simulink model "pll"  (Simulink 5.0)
settings: Solver=ode4  StartTime=0.0  StopTime=5  FixedStep=0.001  RelTol=1e-6
libraries: simulink x1

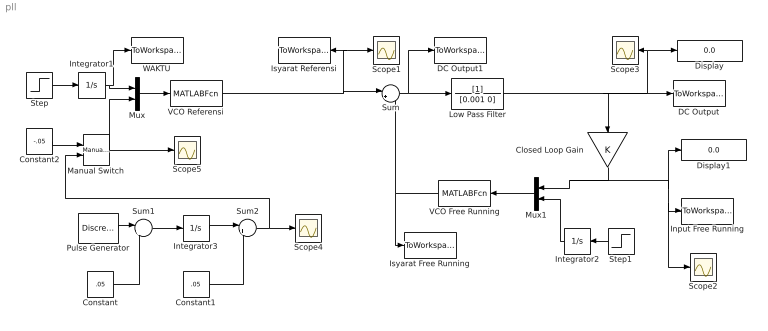
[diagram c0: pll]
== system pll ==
  Closed Loop Gain : Gain  Orientation=down
  Constant : Constant  Value=.05
  Constant1 : Constant  Value=.05
  Constant2 : Constant  Value=-.05
  DC Output : ToWorkspace  VariableName=vout  SampleTime=-1  SaveFormat=Array
  DC Output1 : ToWorkspace  VariableName=outcomp  SampleTime=-1  SaveFormat=Array
  Display : Display
  Display1 : Display
  Input Free Running : ToWorkspace  VariableName=vin  SampleTime=-1  SaveFormat=Array
  Integrator1 : Integrator
  Integrator2 : Integrator  Orientation=left
  Integrator3 : Integrator
  Isyarat Free Running : ToWorkspace  VariableName=frun  SampleTime=-1  SaveFormat=Array
  Isyarat Referensi : ToWorkspace  VariableName=fref  SampleTime=-1  SaveFormat=Array
  Low Pass Filter : TransferFcn  Denominator=[0.001 0]
  Manual Switch : simulink/Signal Routing/Manual Switch  sw=1  action=0
  Mux : Mux  Inputs=2
  Mux1 : Mux  Orientation=left  Inputs=2
  Pulse Generator : DiscretePulseGenerator  PulseType=Time based  Amplitude=0.1  Period=4  PulseWidth=50
  Scope{1..5} (5 alike) : Scope
  Step : Step  Time=0  SampleTime=0
  Step1 : Step  Orientation=left  Time=0  SampleTime=0
  Sum : Sum  Inputs=|+-
  Sum1 : Sum  Inputs=|+-
  Sum2 : Sum  Inputs=|+-
  VCO Free Running : MATLABFcn  Orientation=left  MATLABFcn=vcorun
  VCO Referensi : MATLABFcn  MATLABFcn=vcoref
  WAKTU : ToWorkspace  VariableName=time  SampleTime=-1  SaveFormat=Array
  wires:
  Step/1 -> Integrator1/1
  Integrator1/1 -> Mux/1, WAKTU/1
  Mux/1 -> VCO Referensi/1
  VCO Referensi/1 -> Scope1/1, Isyarat Referensi/1, Sum/1
  VCO Free Running/1 -> Isyarat Free Running/1, Sum/2
  Mux1/1 -> VCO Free Running/1
  Step1/1 -> Integrator2/1
  Integrator2/1 -> Mux1/2
  Low Pass Filter/1 -> DC Output/1, Closed Loop Gain/1, Display/1, Scope3/1
  Closed Loop Gain/1 -> Mux1/1, Display1/1, Input Free Running/1, Scope2/1
  Sum/1 -> DC Output1/1, Low Pass Filter/1
  Pulse Generator/1 -> Sum1/1
  Constant/1 -> Sum1/2
  Sum1/1 -> Integrator3/1
  Integrator3/1 -> Sum2/1
  Constant1/1 -> Sum2/2
  Sum2/1 -> Scope4/1, Manual Switch/2
  Constant2/1 -> Manual Switch/1
  Manual Switch/1 -> Mux/2, Scope5/1
